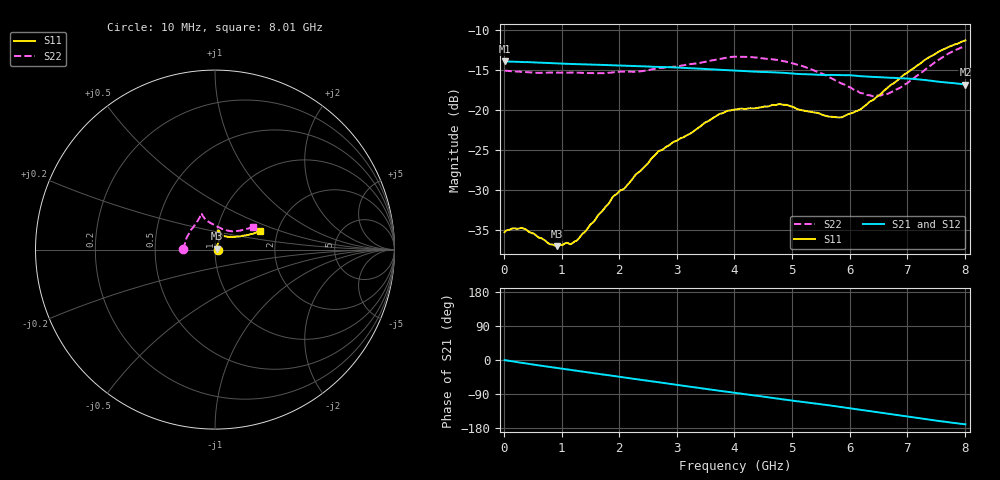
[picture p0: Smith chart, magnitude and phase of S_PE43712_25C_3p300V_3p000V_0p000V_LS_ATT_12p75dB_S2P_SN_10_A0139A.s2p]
! DEVICE ID: PE43712
! File Path: z:\PE43713\PE43713_CHAR_NOM_04292014\AMB\3p300\LS_ATT_12p75dB\PE43713_AMB_3p300V_3p000V_0p000V_LS_ATT_12p75dB_S2P_SN_10_A0139A.s2p
! Serial: 10
! Lot: A0139A
! Temp: 25C
! VDD: 3.300
! VSS: 0.000
! Control_Hi: 3.000
! Control_Lo: 0.000
! Attenuation Step: 12.75dB
! Port 1: RF1
! Port 2: RF2
! ThroughPath:1-2
! IDD: 0.0001470346
! ISS: -1.046e-007
#  Hz  S  RI  R  50
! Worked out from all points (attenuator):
!   801 points, 10 MHz to 8.01 GHz, reference 50 ohm
!   highest |S21| = -13.94 dB at 10 MHz (marker M1); lowest = -16.8 dB at 8.01 GHz (marker M2)
!   lowest |S11| = -37.0 dB at 920 MHz (marker M3), VSWR 1.03, Z = 51.3 + j0.54 ohm
!   |S11| at or under -10 dB: start of sweep to end of sweep
!   |S22| runs from -18.3 to -12.1 dB; largest |S21 - S12| = 0.00073
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1e7  0.0172 0.000298  0.201 -0.00106  0.2011 -0.00101  -0.1762 0.00113
3.4e8  0.0181 0.000339  0.1971 -0.0283  0.1971 -0.0279  -0.1716 0.0202
7.8e8  0.0142 0.0036  0.1868 -0.0611  0.1868 -0.0612  -0.1655 0.0444
9.2e8  0.0131 0.00526  0.1823 -0.0708  0.1824 -0.0709  -0.1632 0.0516
1.18e9  0.0111 0.00948  0.173 -0.0873  0.173 -0.0875  -0.1582 0.0657
1.35e9  0.0113 0.0122  0.1664 -0.0977  0.1664 -0.0977  -0.1539 0.0736
1.9e9  0.0134 0.0256  0.1412 -0.1276  0.1412 -0.1276  -0.1368 0.1044
2.11e9  0.0145 0.0295  0.1301 -0.1375  0.1301 -0.1375  -0.131 0.1137
2.68e9  0.0227 0.0502  0.0966 -0.1586  0.0965 -0.1586  -0.1061 0.149
3.72e9  0.0233 0.0904  0.0288 -0.1762  0.0287 -0.1762  -0.0825 0.1905
4.01e9  0.0218 0.0983  0.00992 -0.1762  0.0099 -0.1762  -0.0822 0.1989
4.79e9  0.0196 0.107  -0.0376 -0.1668  -0.0376 -0.167  -0.0705 0.1916
5.35e9  0.03 0.0922  -0.0676 -0.1525  -0.0675 -0.1524  -0.0556 0.17
5.64e9  0.0403 0.0815  -0.0816 -0.1441  -0.0816 -0.1441  -0.0369 0.1563
5.88e9  0.051 0.0747  -0.0942 -0.1357  -0.0939 -0.1357  -0.0174 0.1447
6.17e9  0.07 0.0714  -0.1071 -0.1226  -0.1069 -0.1228  0.0115 0.1282
6.38e9  0.0887 0.0717  -0.1147 -0.1132  -0.1145 -0.1132  0.0349 0.1174
6.68e9  0.12 0.0718  -0.125 -0.0985  -0.1247 -0.0985  0.0712 0.1054
7e9  0.1528 0.0766  -0.1344 -0.0815  -0.1342 -0.0814  0.1059 0.102
7.36e9  0.1934 0.085  -0.1407 -0.0601  -0.1405 -0.0601  0.1488 0.1085
7.72e9  0.2291 0.0948  -0.1425 -0.04  -0.1424 -0.0402  0.1911 0.1202
8.01e9  0.2504 0.1061  -0.1418 -0.0255  -0.1416 -0.0258  0.2129 0.1276
